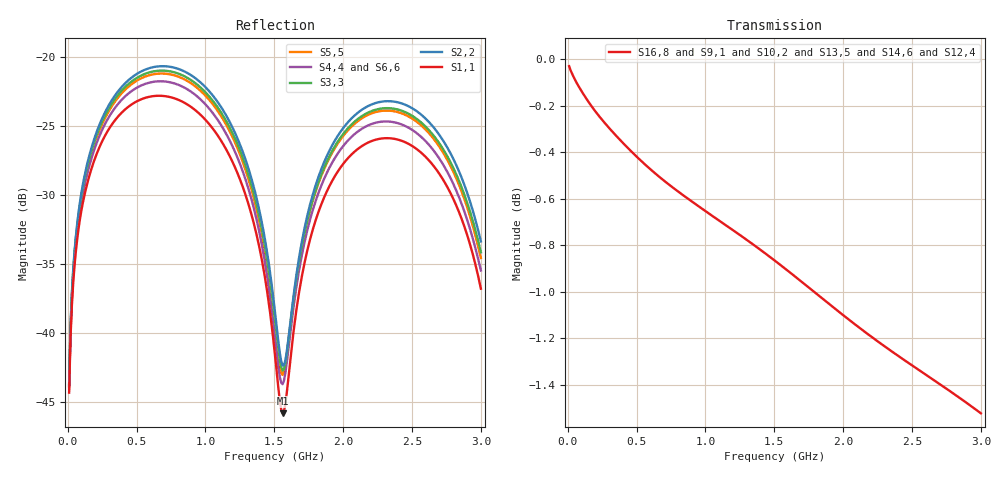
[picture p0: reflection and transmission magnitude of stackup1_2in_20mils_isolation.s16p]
! Touchstone file from project
# GHZ S RI R 50.000000
! Modal data exported
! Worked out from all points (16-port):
!   300 points, 10 MHz to 3 GHz, reference 50 ohm
!   strongest paths, dB at 10 MHz, 760 MHz, 1.51 GHz, 2.26 GHz, 3 GHz:
!     S16,8: 0.0, -0.5, -0.9, -1.2, -1.5
!     S9,1: 0.0, -0.6, -0.9, -1.2, -1.5
!     S10,2: 0.0, -0.6, -0.9, -1.2, -1.6
!     S13,5: 0.0, -0.6, -0.9, -1.2, -1.6
!     S14,6: 0.0, -0.6, -0.9, -1.2, -1.6
!     S12,4: 0.0, -0.6, -0.9, -1.2, -1.6
!   lowest |S11| = -45.8 dB at 1.56 GHz (marker M1), VSWR 1.01, Z = 50.5 - j0.166 ohm
!   |S11| at or under -10 dB: start of sweep to end of sweep
